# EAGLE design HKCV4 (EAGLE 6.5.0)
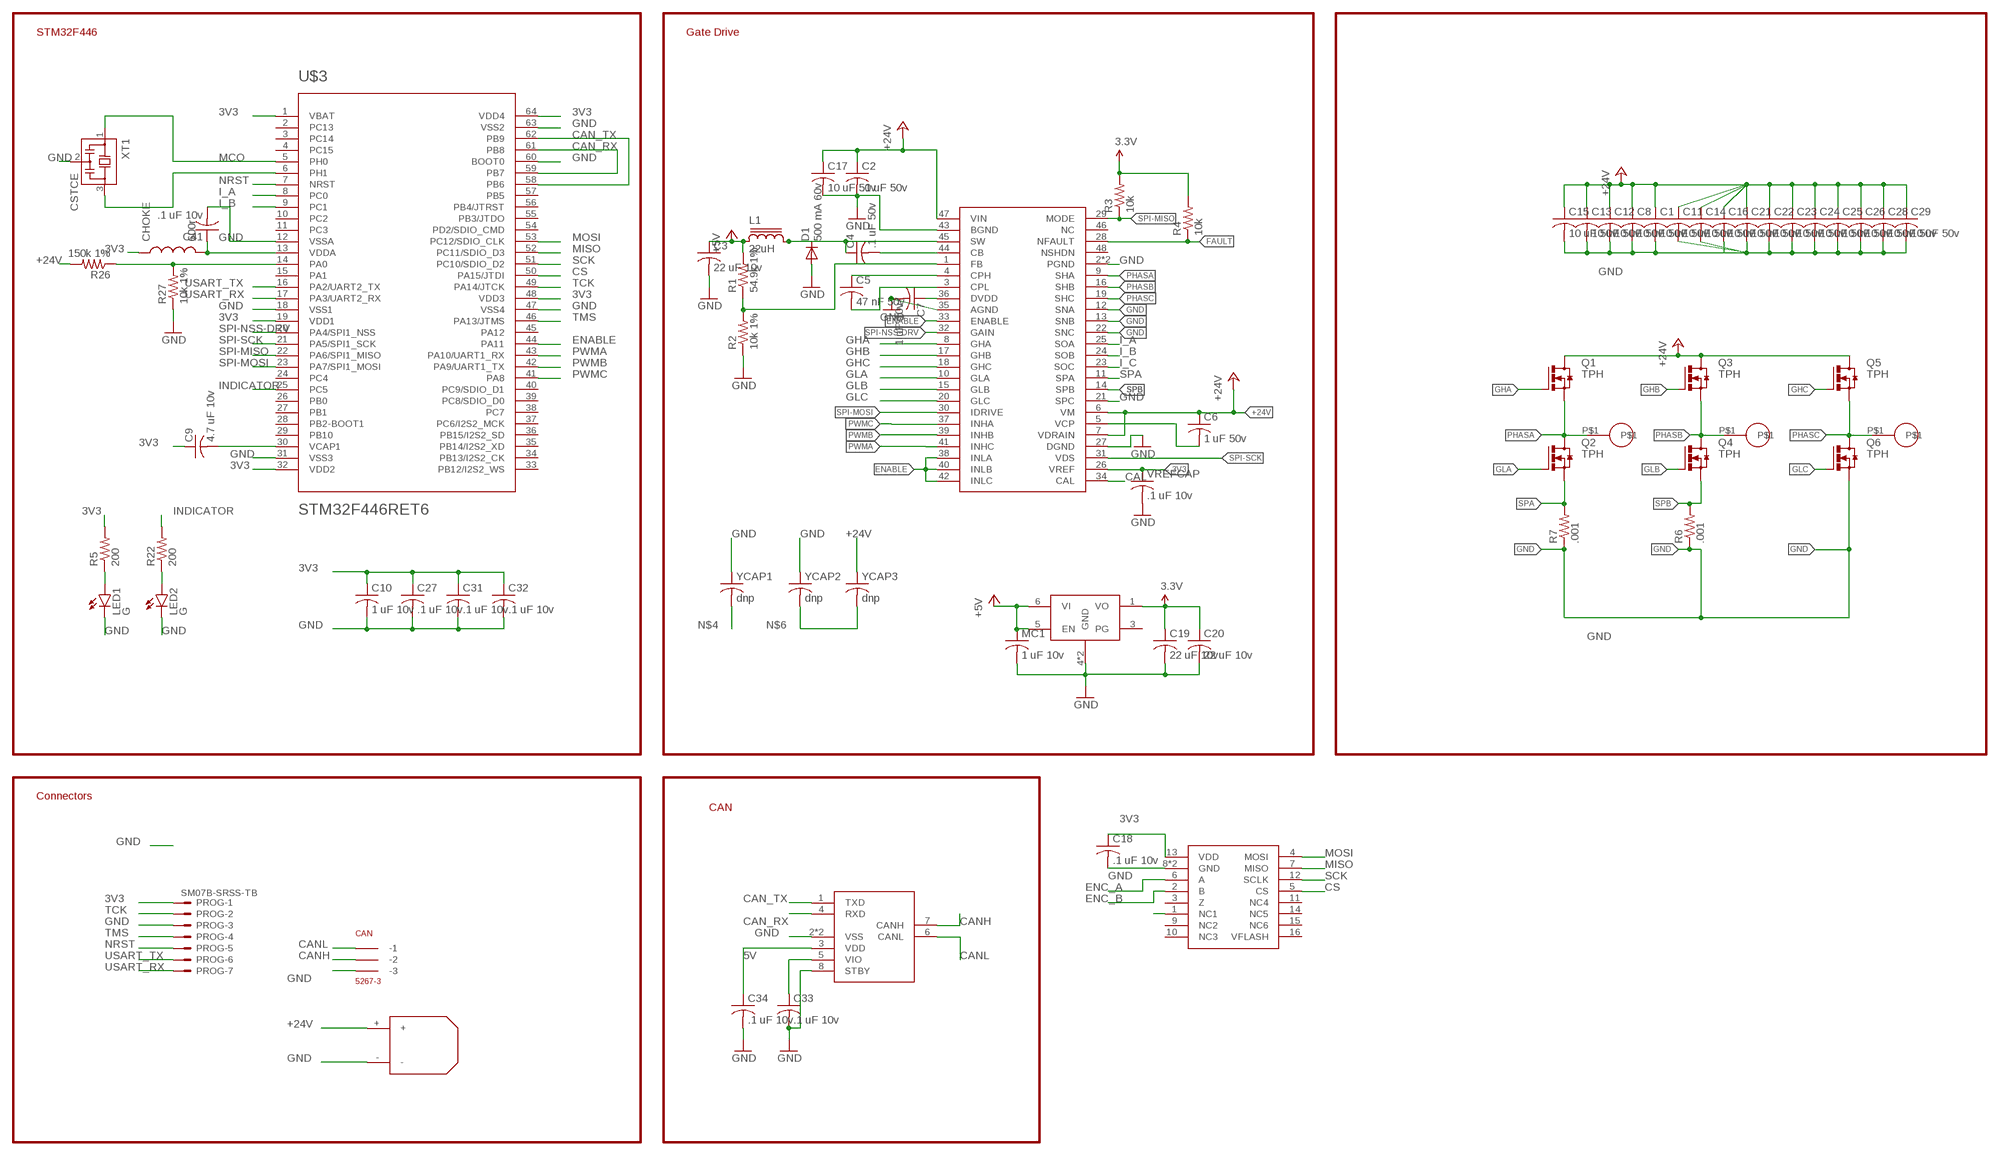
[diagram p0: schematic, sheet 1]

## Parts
C1  10 uF 50v  C-USC1206K  [C1206K]
C2  .1 uF 50v  C-USC0603K  [C0603K]
C3  22 uF 10v  C-USC0603K  [C0603K]
C4  .1 uF 50v  C-USC0603K  [C0603K]
C5  47 nF 50v  C-USC0402K  [C0402K]
C6  1 uF 50v  C-USC0603K  [C0603K]
C7  1 uF 10v  C-USC0402K  [C0402K]
C8  10 uF 50v  C-USC1206K  [C1206K]
C9  4.7 uF 10v  C-USC0402K  [C0402K]
C10  1 uF 10v  C-USC0402K  [C0402K]
C11  10 uF 50v  C-USC1206K  [C1206K]
C12  10 uF 50v  C-USC1206K  [C1206K]
C13  10 uF 50v  C-USC1206K  [C1206K]
C14  10 uF 50v  C-USC1206K  [C1206K]
C15  10 uF 50v  C-USC1206K  [C1206K]
C16  10 uF 50v  C-USC1206K  [C1206K]
C17  10 uF 50v  C-USC1206K  [C1206K]
C18  .1 uF 10v  C-USC0402K  [C0402K]
C19  22 uF 10v  C-USC0603K  [C0603K]
C20  22 uF 10v  C-USC0603K  [C0603K]
C21  10 uF 50v  C-USC1206K  [C1206K]
C22  10 uF 50v  C-USC1206K  [C1206K]
C23  10 uF 50v  C-USC1206K  [C1206K]
C24  10 uF 50v  C-USC1206K  [C1206K]
C25  10 uF 50v  C-USC1206K  [C1206K]
C26  10 uF 50v  C-USC1206K  [C1206K]
C27  .1 uF 10v  C-USC0402K  [C0402K]
C28  10 uF 50v  C-USC1206K  [C1206K]
C29  10 uF 50v  C-USC1206K  [C1206K]
C31  .1 uF 10v  C-USC0402K  [C0402K]
C32  .1 uF 10v  C-USC0402K  [C0402K]
C33  .1 uF 10v  C-USC0402K  [C0402K]
C34  .1 uF 10v  C-USC0402K  [C0402K]
C41  .1 uF 10v  C-USC0402K  [C0402K]
CAN  5267-3  [5267-3]
CHOKE  600r  INDUCTOR0603  [0603]
D1  500 mA 60v  DIODE-SOD123  [SOD123]
L1  22uH  SDR0302  [SDR0302]
LDFM33PUR  LDFM  [DFN6-3X3]
LED1  G  LED0603  [LED-0603]
LED2  G  LED0603  [LED-0603]
MC1  1 uF 10v  C-USC0402K  [C0402K]
PROG  SM07B-SRSS-TB  [SM07B-SRSS-TB]
Q1  TPH  [TRANS_TPH5900CNH,L1Q]
Q2  TPH  [TRANS_TPH5900CNH,L1Q]
Q3  TPH  [TRANS_TPH5900CNH,L1Q]
Q4  TPH  [TRANS_TPH5900CNH,L1Q]
Q5  TPH  [TRANS_TPH5900CNH,L1Q]
Q6  TPH  [TRANS_TPH5900CNH,L1Q]
R1  54.9k 1%  R-US_R0402  [R0402]
R2  10k 1%  R-US_R0402  [R0402]
R3  10k  R-US_R0402  [R0402]
R4  10k  R-US_R0402  [R0402]
R5  200  R-US_R0402  [R0402]
R6  .001  R-US_R1210  [R1210]
R7  .001  R-US_R1210  [R1210]
R22  200  R-US_R0402  [R0402]
R26  150k 1%  R-US_R0402  [R0402]
R27  10k 1%  R-US_R0402  [R0402]
U$1  DRV8323RH  [QFN50P700X700X90-49N]
U$2  18_AWG_PAD  [18_AWG_PAD]
U$3  STM32F446RET6  [TQFP64]
U$4  18_AWG_PAD  [18_AWG_PAD]
U$5  18_AWG_PAD  [18_AWG_PAD]
U$6  MCP2542  [TDFN]
U$9  XT30  [XT30_HORIZONTAL]
U$11  MA700  [QFN16]
VREFCAP  .1 uF 10v  C-USC0402K  [C0402K]
XT1  CSTCE  [CSTCE]
YCAP1  dnp  C-USC0402K  [C0402K]
YCAP2  dnp  C-USC0402K  [C0402K]
YCAP3  dnp  C-USC0402K  [C0402K]

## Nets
3V3: C9.1 C10.1 C18.1 C19.1 C20.1 C27.1 C31.1 C32.1 C33.1 CHOKE.1 LDFM33PUR.1(VO) PROG.1 R3.2 R4.2 R5.2 U$1.26(VREF) U$3.1(VBAT) U$3.19(VDD1) U$3.32(VDD2) U$3.48(VDD3) U$3.64(VDD4) U$6.5(VIO) U$11.13(VDD) VREFCAP.1 ; supply symbol labelled 3.3V
5V: C3.1 C34.1 L1.1 LDFM33PUR.5(EN) LDFM33PUR.6(VI) MC1.1 R1.2 U$6.3(VDD) ; supply symbol labelled +5V
+24V: C1.1 C2.1 C6.1 C8.1 C11.1 C12.1 C13.1 C14.1 C15.1 C16.1 C17.1 C21.1 C22.1 C23.1 C24.1 C25.1 C26.1 C28.1 C29.1 Q1.5(D) Q1.6(D) Q1.7(D) Q1.8(D) Q1.EP(D) Q3.5(D) Q3.6(D) Q3.7(D) Q3.8(D) Q3.EP(D) Q5.5(D) Q5.6(D) Q5.7(D) Q5.8(D) Q5.EP(D) R26.2 U$1.6(VM) U$1.7(VDRAIN) U$1.47(VIN) U$9.+ YCAP3.1
BOOT: C4.2 U$1.44(CB)
CAL: U$1.34(CAL)
CAN_RX: U$3.59(PB7) U$3.61(PB8) U$6.4(RXD)
CAN_TX: U$3.58(PB6) U$3.62(PB9) U$6.1(TXD)
CANH: CAN.P$2(-2) U$6.7(CANH)
CANL: CAN.P$1(-1) U$6.6(CANL)
CPH: C5.1 U$1.4(CPH)
CPL: C5.2 U$1.3(CPL)
CS: U$3.50(PA15/JTDI) U$11.5(CS)
DEVICE3.3: C7.1 U$1.36(DVDD)
ENABLE: U$1.33(ENABLE) U$1.38(INLA) U$1.40(INLB) U$1.42(INLC) U$3.44(PA11)
ENC_A: U$11.6(A)
ENC_B: U$11.2(B)
FAULT: R4.1 U$1.28(NFAULT)
FB: R1.1 R2.2 U$1.1(FB)
GHA: Q1.4(G) U$1.8(GHA)
GHB: Q3.4(G) U$1.17(GHB)
GHC: Q5.4(G) U$1.18(GHC)
GLA: Q2.4(G) U$1.10(GLA)
GLB: Q4.4(G) U$1.15(GLB)
GLC: Q6.4(G) U$1.20(GLC)
GND: C1.2 C2.2 C3.2 C7.2 C8.2 C10.2 C11.2 C12.2 C13.2 C14.2 C15.2 C16.2 C17.2 C18.2 C19.2 C20.2 C21.2 C22.2 C23.2 C24.2 C25.2 C26.2 C27.2 C28.2 C29.2 C31.2 C32.2 C33.2 C34.2 C41.2 CAN.P$3(-3) D1.A LDFM33PUR.4(GND) LDFM33PUR.EXP(GND) LED1.C LED2.C MC1.2 PROG.3 Q6.1(S) Q6.2(S) Q6.3(S) R2.1 R6.1 R7.1 R27.1 U$1.2(PGND) U$1.12(SNA) U$1.13(SNB) U$1.21(SPC) U$1.22(SNC) U$1.27(DGND) U$1.35(AGND) U$1.43(BGND) U$1.49(PGND) U$3.12(VSSA) U$3.18(VSS1) U$3.31(VSS3) U$3.47(VSS4) U$3.60(BOOT0) U$3.63(VSS2) U$6.2(VSS) U$6.8(STBY) U$6.9(VSS) U$9.- U$11.8(GND) U$11.TH(GND) VREFCAP.2 XT1.2 YCAP1.1 YCAP2.1
I_A: U$1.25(SOA) U$3.8(PC0)
I_B: U$1.24(SOB) U$3.9(PC1)
I_C: U$1.23(SOC)
INDICATOR: R22.2 U$3.25(PC5)
MCO: U$3.5(PH0) XT1.1
MISO: U$3.52(PC11/SDIO_D3) U$11.7(MISO)
MOSI: U$3.53(PC12/SDIO_CLK) U$11.4(MOSI)
N$1: LED1.A R5.1
N$2: C41.1 CHOKE.2 U$3.13(VDDA)
N$3: C9.2 U$3.30(VCAP1)
N$4: YCAP1.2
N$6: YCAP2.2 YCAP3.2
N$9: U$11.1(NC1)
N$24: R26.1 R27.2 U$3.14(PA0)
N$28: LED2.A R22.1
N$30: U$3.6(PH1) XT1.3
NRST: PROG.5 U$3.7(NRST)
PHASA: Q1.1(S) Q1.2(S) Q1.3(S) Q2.5(D) Q2.6(D) Q2.7(D) Q2.8(D) Q2.EP(D) U$1.9(SHA) U$4.P$1
PHASB: Q3.1(S) Q3.2(S) Q3.3(S) Q4.5(D) Q4.6(D) Q4.7(D) Q4.8(D) Q4.EP(D) U$1.16(SHB) U$2.P$1
PHASC: Q5.1(S) Q5.2(S) Q5.3(S) Q6.5(D) Q6.6(D) Q6.7(D) Q6.8(D) Q6.EP(D) U$1.19(SHC) U$5.P$1
PWMA: U$1.41(INHC) U$3.43(PA10/UART1_RX)
PWMB: U$1.39(INHB) U$3.42(PA9/UART1_TX)
PWMC: U$1.37(INHA) U$3.41(PA8)
SCK: U$3.51(PC10/SDIO_D2) U$11.12(SCLK)
SPA: Q2.1(S) Q2.2(S) Q2.3(S) R7.2 U$1.11(SPA)
SPB: Q4.1(S) Q4.2(S) Q4.3(S) R6.2 U$1.14(SPB)
SPI-MISO: R3.1 U$1.29(MODE) U$3.22(PA6/SPI1_MISO)
SPI-MOSI: U$1.30(IDRIVE) U$3.23(PA7/SPI1_MOSI)
SPI-NSS-DRV: U$1.32(GAIN) U$3.20(PA4/SPI1_NSS)
SPI-SCK: U$1.31(VDS) U$3.21(PA5/SPI1_SCK)
SW: C4.1 D1.C L1.2 U$1.45(SW)
TCK: PROG.2 U$3.49(PA14/JTCK)
TMS: PROG.4 U$3.46(PA13/JTMS)
USART_RX: PROG.7 U$3.17(PA3/UART2_RX)
USART_TX: PROG.6 U$3.16(PA2/UART2_TX)
VCP: C6.2 U$1.5(VCP)
Unconnected: LDFM33PUR.3(PG) U$1.46(NC) U$1.48(NSHDN) U$3.2(PC13) U$3.3(PC14) U$3.4(PC15) U$3.10(PC2) U$3.11(PC3) U$3.15(PA1) U$3.24(PC4) U$3.26(PB0) U$3.27(PB1) U$3.28(PB2-BOOT1) U$3.29(PB10) U$3.33(PB12/I2S2_WS) U$3.34(PB13/I2S2_CK) U$3.35(PB14/I2S2_XD) U$3.36(PB15/I2S2_SD) U$3.37(PC6/I2S2_MCK) U$3.38(PC7) U$3.39(PC8/SDIO_D0) U$3.40(PC9/SDIO_D1) U$3.45(PA12) U$3.54(PD2/SDIO_CMD) U$3.55(PB3/JTDO) U$3.56(PB4/JTRST) U$3.57(PB5) U$11.3(Z) U$11.9(NC2) U$11.10(NC3) U$11.11(NC4) U$11.14(NC5) U$11.15(NC6) U$11.16(VFLASH)

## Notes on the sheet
- STM32F446 | Gate Drive
- Connectors
- CAN

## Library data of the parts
C1-C29 C31-C34 C41 MC1 VREFCAP YCAP1-YCAP3 = rcl:C-US: CAPACITOR, American symbol
CAN = con-molex-spox:5267-3
CHOKE = SparkFun-Passives:INDUCTOR: Inductors
D1 = diode:DIODE-: DIODE
L1 = inductor-bourns:SDR0302: POWER INDUCTOR
LDFM33PUR = BenLibrary:LDFM
LED1 LED2 = SparkFun-LED:LED: LEDs
PROG = con-jst2:?M07B-SRSS-TB: Disconnectable Crimp style connector, 1.0mm pitch 7 contacts
Q1-Q6 = transistor-power:TPH
R1-R7 R22 R26 R27 = rcl:R-US_: RESISTOR, American symbol
U$1 = BenLibrary:DRV8323RH
U$2 U$4 U$5 = BenLibrary:18_AWG_PAD
U$3 = BenLibrary:STM32F446RET6: ARM DSP Chip used on the WAV Trigger board.
U$6 = BenLibrary:MCP2542
U$9 = Ben_Library:XT30
U$11 = BenLibrary:MA700
XT1 = sc_usercreated:CSTCE

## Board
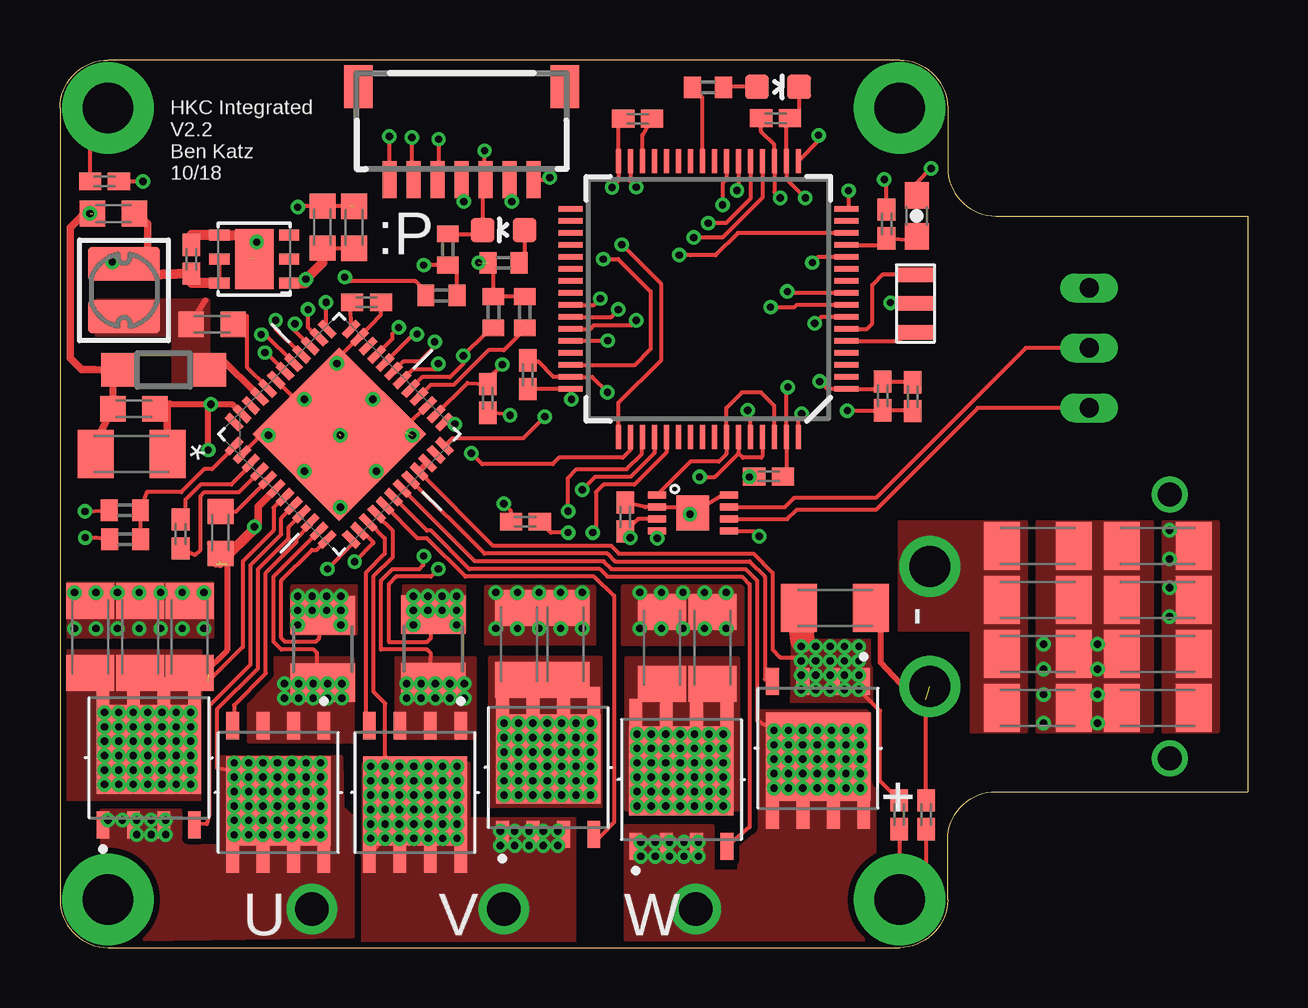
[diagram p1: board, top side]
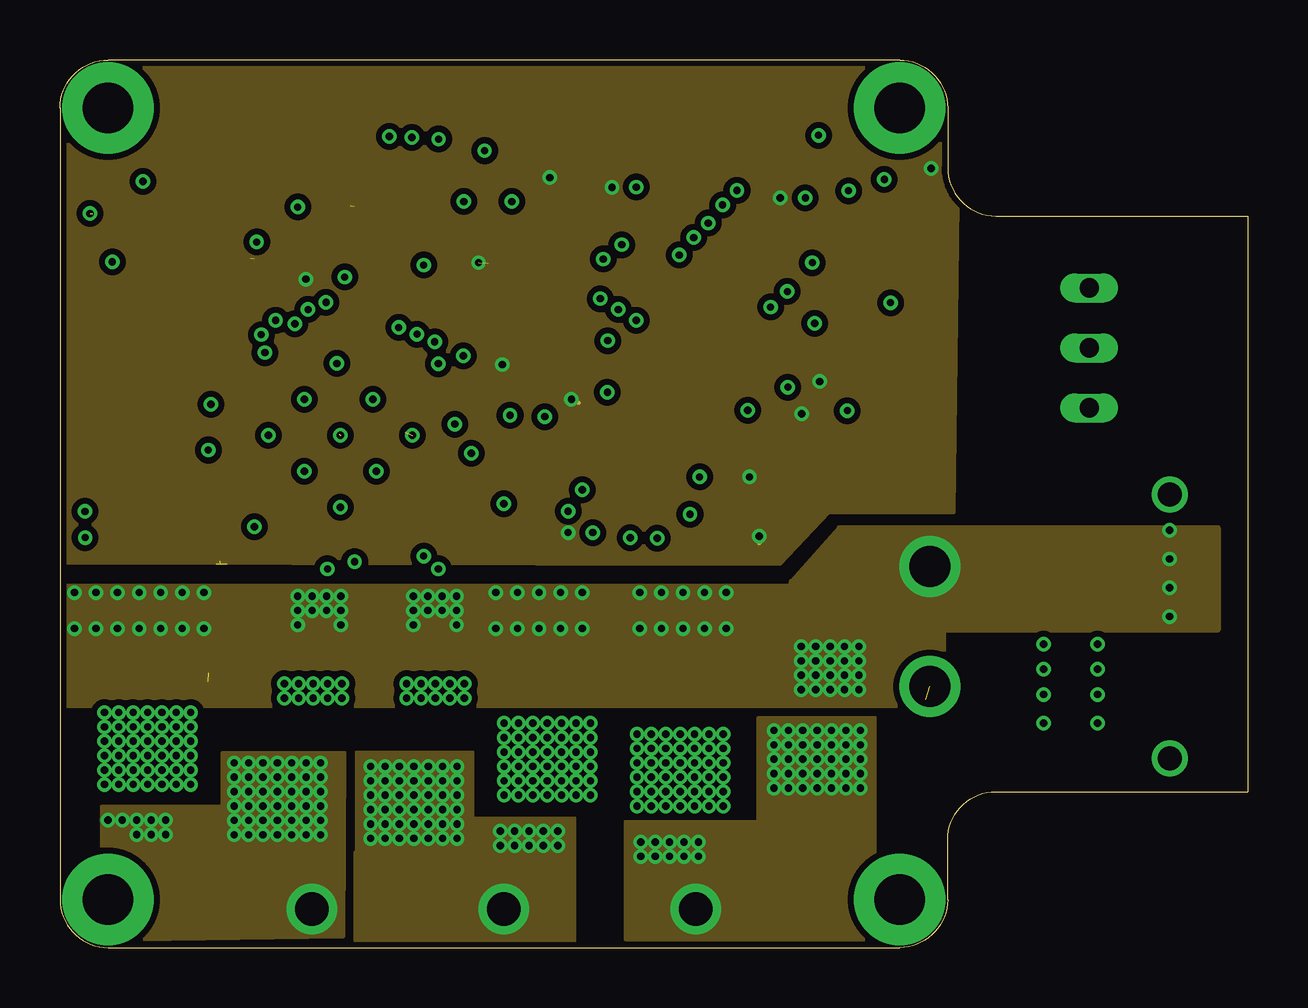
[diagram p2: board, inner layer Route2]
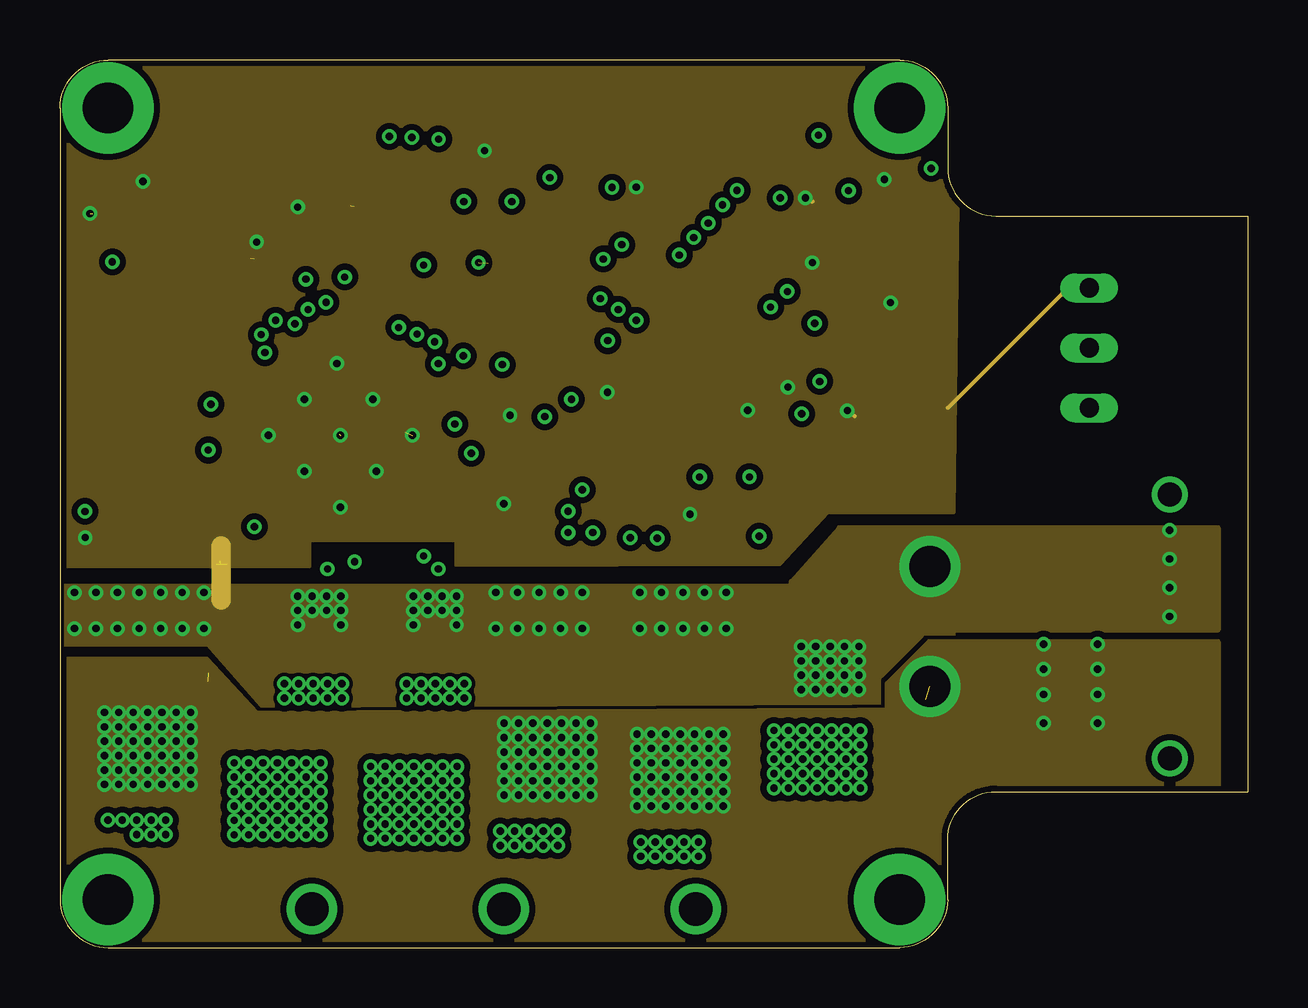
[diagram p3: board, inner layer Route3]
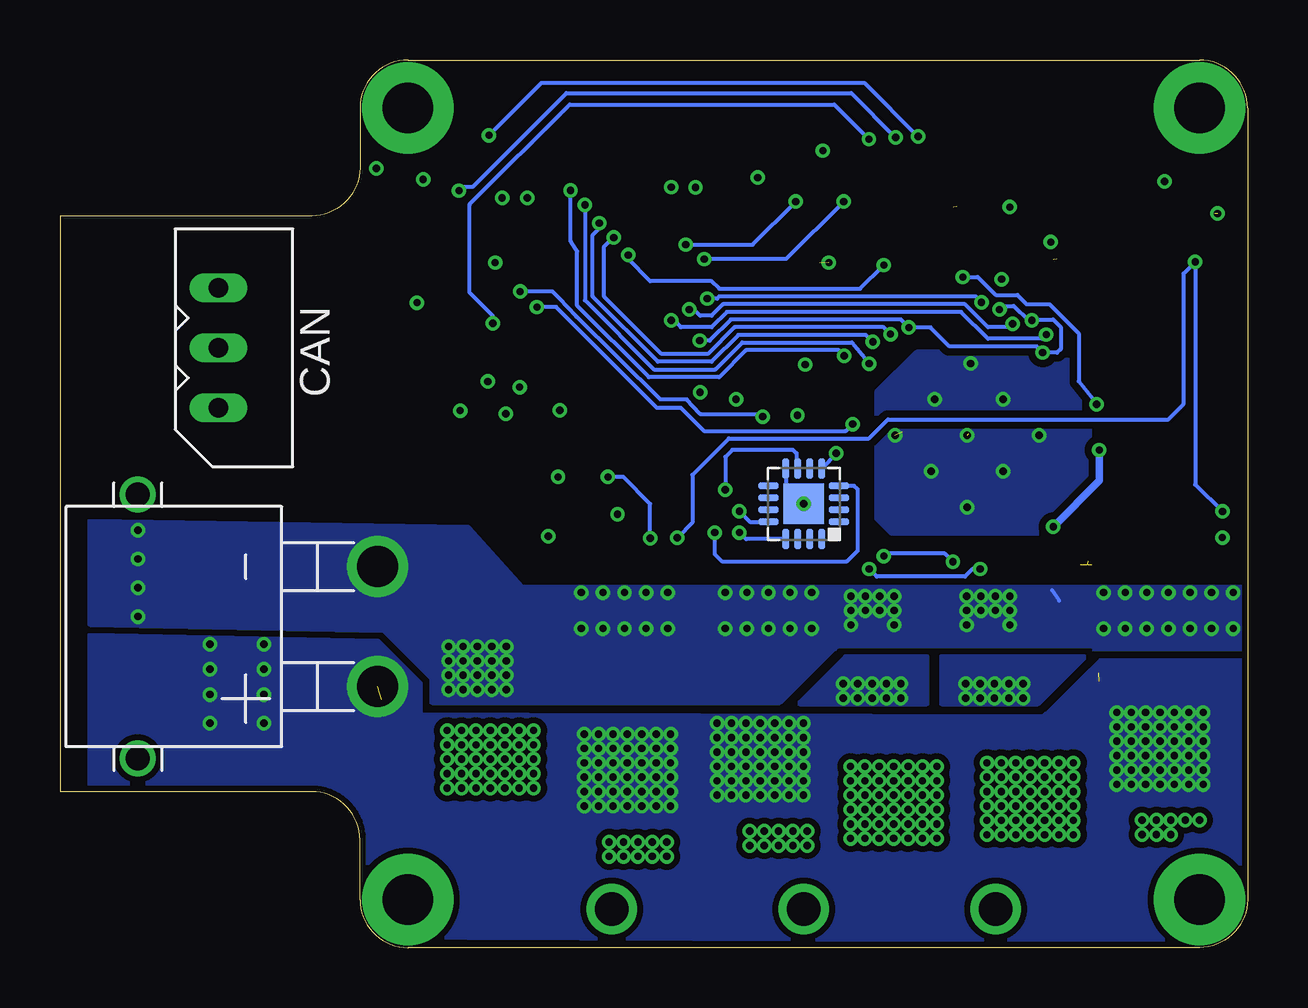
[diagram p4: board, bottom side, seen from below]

Size 49.5 x 37 mm. Coordinates in mm from the lower left corner, seen from the top.
Outline: 2,0 35,0 arc90 37,2 37,4.5 arc-90 39,6.5 49.5,6.5 49.5,30.5 39,30.5 arc-90 37,32.5 37,35 arc90 35,37 2,37 arc90 0,35 0,2 arc90 2,0
Copper layers (1*2+3*16): Top 0.035mm / dielectric 1.5mm / Route2 0.035mm / dielectric 0.15mm / Route3 0.035mm / dielectric 0.2mm / Bottom 0.035mm
Design rules "default *": minimum track width 6mil, minimum drill 0.3mm, track to track 6mil, track to pad 6mil, pad to pad 6mil, via to via 6mil, smd to smd 6mil, copper to edge 6mil, drill to drill 6mil, minimum pad ring 0.15mm, minimum via ring 0.15mm, stop-mask expansion 4mil, vias tented up to drill 12mil, thermal gap 10mil

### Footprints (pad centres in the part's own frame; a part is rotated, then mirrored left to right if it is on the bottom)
C1206K = smd 1.5 x 2: 1 -1.5,0; 2 1.5,0
C0603K = smd 1.05 x 1.08: 1 -0.875,0; 2 0.875,0
C0402K = smd 0.925 x 0.74: 1 -0.6,0; 2 0.6,0
5267-3 = drill 0.8 long: P$1 0,0; P$2 2.5,0; P$3 5,0
0603 = smd 1.1 x 1: 1 -0.85,0; 2 0.85,0
SOD123 = smd 1.4 x 1.4: A 1.9,0; C -1.9,0
SDR0302 = smd 3 x 1.4: 1 0,1.1; 2 0,-1.1
DFN6-3X3 = smd 0.85 x 0.45: 1 -1.45,1; 2 -1.45,0; 3 -1.45,-1; 4 1.45,-1; 5 1.45,0; 6 1.45,1 | smd 1.6 x 2.5: EXP 0,0
LED-0603 = smd 1 x 1: A 0,-0.877; C 0,0.877
SM07B-SRSS-TB = smd 0.6 x 1.55: 1 -3,2.975; 2 -2,2.975; 3 -1,2.975; 4 0,2.975; 5 1,2.975; 6 2,2.975; 7 3,2.975 | smd 1.2 x 1.8: FIT@1 -4.3,-0.9; FIT@2 4.3,-0.9
TRANS_TPH5900CNH,L1Q = smd 1.13 x 0.53: 1 -2.79,1.905; 2 -2.79,0.635; 3 -2.79,-0.635; 4 -2.79,-1.905 | smd 1.33 x 0.53: 5 2.69,-1.905; 6 2.69,-0.635; 7 2.69,0.635; 8 2.69,1.905 | smd 3.7 x 4.35: EP 0.35,0
R0402 = smd 0.7 x 0.9: 1 -0.65,0; 2 0.65,0
R1210 = smd 1.6 x 2.7: 1 -1.4,0; 2 1.4,0
QFN50P700X700X90-49N = smd 0.813 x 0.305: 1 -3.454,2.743; 2 -3.454,2.261; 3 -3.454,1.753; 4 -3.454,1.245; 5 -3.454,0.762; 6 -3.454,0.254; 7 -3.454,-0.254; 8 -3.454,-0.762; 9 -3.454,-1.245; 10 -3.454,-1.753; 11 -3.454,-2.261; 12 -3.454,-2.743; 25 3.454,-2.743; 26 3.454,-2.261; 27 3.454,-1.753; 28 3.454,-1.245; 29 3.454,-0.762; 30 3.454,-0.254; 31 3.454,0.254; 32 3.454,0.762; 33 3.454,1.245; 34 3.454,1.753; 35 3.454,2.261; 36 3.454,2.743 | smd 0.305 x 0.813: 13 -2.743,-3.454; 14 -2.261,-3.454; 15 -1.753,-3.454; 16 -1.245,-3.454; 17 -0.762,-3.454; 18 -0.254,-3.454; 19 0.254,-3.454; 20 0.762,-3.454; 21 1.245,-3.454; 22 1.753,-3.454; 23 2.261,-3.454; 24 2.743,-3.454; 37 2.743,3.454; 38 2.261,3.454; 39 1.753,3.454; 40 1.245,3.454; 41 0.762,3.454; 42 0.254,3.454; 43 -0.254,3.454; 44 -0.762,3.454; 45 -1.245,3.454; 46 -1.753,3.454; 47 -2.261,3.454; 48 -2.743,3.454 | smd 5.105 x 5.105: 49 0,0
18_AWG_PAD = drill 1.4: P$1 0,0
TQFP64 = smd 0.22 x 1: 1 -3.75,-5.75; 2 -3.25,-5.75; 3 -2.75,-5.75; 4 -2.25,-5.75; 5 -1.75,-5.75; 6 -1.25,-5.75; 7 -0.75,-5.75; 8 -0.25,-5.75; 9 0.25,-5.75; 10 0.75,-5.75; 11 1.25,-5.75; 12 1.75,-5.75; 13 2.25,-5.75; 14 2.75,-5.75; 15 3.25,-5.75; 16 3.75,-5.75; 33 3.75,5.75; 34 3.25,5.75; 35 2.75,5.75; 36 2.25,5.75; 37 1.75,5.75; 38 1.25,5.75; 39 0.75,5.75; 40 0.25,5.75; 41 -0.25,5.75; 42 -0.75,5.75; 43 -1.25,5.75; 44 -1.75,5.75; 45 -2.25,5.75; 46 -2.75,5.75; 47 -3.25,5.75; 48 -3.75,5.75 | smd 1 x 0.22: 17 5.75,-3.75; 18 5.75,-3.25; 19 5.75,-2.75; 20 5.75,-2.25; 21 5.75,-1.75; 22 5.75,-1.25; 23 5.75,-0.75; 24 5.75,-0.25; 25 5.75,0.25; 26 5.75,0.75; 27 5.75,1.25; 28 5.75,1.75; 29 5.75,2.25; 30 5.75,2.75; 31 5.75,3.25; 32 5.75,3.75; 49 -5.75,3.75; 50 -5.75,3.25; 51 -5.75,2.75; 52 -5.75,2.25; 53 -5.75,1.75; 54 -5.75,1.25; 55 -5.75,0.75; 56 -5.75,0.25; 57 -5.75,-0.25; 58 -5.75,-0.75; 59 -5.75,-1.25; 60 -5.75,-1.75; 61 -5.75,-2.25; 62 -5.75,-2.75; 63 -5.75,-3.25; 64 -5.75,-3.75
TDFN = smd 0.3 x 0.75: 1 0,-3; 2 0.5,-3; 3 1,-3; 4 1.5,-3; 5 1.5,0; 6 1,0; 7 0.5,0; 8 0,0 | smd 1.46 x 1.36: 9 0.75,-1.5
XT30_HORIZONTAL = drill 1.7: + -2.5,0; - 2.5,0 | drill 1: P$3 5.5,10; P$4 -5.5,10
QFN16 = smd 0.85 x 0.3: 1 -1.475,0.75; 2 -1.475,0.25; 3 -1.475,-0.25; 4 -1.475,-0.75; 9 1.475,-0.75; 10 1.475,-0.25; 11 1.475,0.25; 12 1.475,0.75 | smd 0.3 x 0.85: 5 -0.75,-1.475; 6 -0.25,-1.475; 7 0.25,-1.475; 8 0.75,-1.475; 13 0.75,1.475; 14 0.25,1.475; 15 -0.25,1.475; 16 -0.75,1.475 | smd 1.7 x 1.7: TH 0,0
CSTCE = smd 0.6 x 1.6: 1 -1.2,0; 2 0,0; 3 1.2,0

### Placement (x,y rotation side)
C1  19.13,12.65 90 top
C2  3.08,22.46 180 top
C3  2.23,30.59 180 top
C4  6.34,25.98 0 top
C5  5.03,17.24 90 top
C6  6.69,17.3 90 top
C7  12.78,26.9 0 top
C8  5.4,12.95 90 top
C9  24.08,34.55 0 top
C10  35.54,22.96 270 top
C11  3.35,12.95 90 top
C12  27.19,12.5 90 top
C13  25.09,12.5 90 top
C14  21.07,12.65 90 top
C15  1.25,12.95 90 top
C16  32.31,14.15 180 top
C17  2.98,20.58 180 top
C18  19.4,17.75 180 top
C19  10.94,30.03 90 top
C20  12.26,30.02 90 top
C21  45.75,14.5 0 top
C22  40.75,16.75 180 top
C23  40.75,14.5 180 top
C24  40.75,12.25 180 top
C25  40.75,10 180 top
C26  45.75,16.75 0 top
C27  29.83,34.57 0 top
C28  45.75,12.25 0 top
C29  45.75,10 0 top
C31  34.29,23 270 top
C32  19.5,23.88 90 top
C33  29.54,19.64 0 top
C34  23.56,17.95 90 top
C41  34.45,30.16 90 top
CAN  42.9,22.5 90 bottom
CHOKE  35.71,30.5 270 top
D1  4.32,24.08 180 top
L1  2.67,27.4 0 top
LDFM33PUR  8.1,28.7 180 top
LED1  18.49,29.91 90 top
LED2  29.93,35.88 270 top
MC1  5.48,28.69 90 top
PROG  16.74,34.98 180 top
Q1  3.7,7.91 90 top
Q2  9.1,6.46 270 top
Q3  20.35,7.51 90 top
Q4  14.8,6.46 270 top
Q5  25.9,7.01 90 top
Q6  31.6,8.31 270 top
R1  2.7,18.23 180 top
R2  2.72,17.02 0 top
R3  18.07,26.48 90 top
R4  19.38,26.48 90 top
R5  18.49,28.54 180 top
R6  15.56,12.47 270 top
R7  10.96,12.45 270 top
R22  27.01,35.85 180 top
R26  15.9,27.18 180 top
R27  16.17,29.1 270 top
U$1  11.64,21.4 45 top
U$2  18.5,1.6 0 top
U$3  27.03,27.04 90 top
U$4  10.5,1.6 0 top
U$5  26.5,1.6 0 top
U$6  27.88,18.86 270 top
U$9  36.26,13.38 90 bottom
U$11  18.5,18.5 180 bottom
VREFCAP  17.83,22.89 270 top
XT1  35.66,26.85 90 top
YCAP1  1.86,31.94 180 top
YCAP2  34.98,5.54 270 top
YCAP3  36.1,5.54 270 top

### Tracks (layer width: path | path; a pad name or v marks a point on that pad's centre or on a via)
3V3  (via drill 0.3)  (1 unrouted)
  Top 0.16: R4.2 R3.2 18.07,28.31 R5.2 | v21.32,22.85 21.28,22.89 U$3.48 C32.1 | U$3.64 30.78,22.11 v30.92,22.25 | v31.67,23.6 31.98,23.29 U$3.1 34.29,23.29 C31.1 35.54,23.6 C10.1 | v30.02,31.25 29.78,31.49 U$3.19 29.78,33.46 29.22,34.02 C27.1 | U$6.5 28.94,17.36 v29.15,17.15 | v21.18,17.3 20.45,17.3 C18.1 | CHOKE.1 35.71,31.88 v36.31,32.48 | 28.72,19.62 v28.74,19.62 28.76,19.64 C33.1 | C9.1 23.28,34.31 U$3.32 23.28,31.96 v23.01,31.69 | U$1.26 16.98,23.54 VREFCAP.1 17.83,23.69 v18.44,24.3 | C20.1 C19.1 | PROG.1 20.42,32.01 v20.42,32.1
  Top 0.406: LDFM33PUR.1 10.25,27.7 v10.25,27.86 10.94,28.55 C19.1
  Route2 0.16: v21.32,22.85 21.47,22.85 21.62,22.7 | v30.92,22.25 31.07,22.4 | v31.67,23.6 31.67,23.75 | v30.02,31.25 30.17,31.1 | v29.15,17.15 29.15,16.85
  Bottom 0.16: U$11.13 20.91,17.02 v21.18,17.3
  other vias: 17.45,28.55
  pour Route2 (isolate 0.254, no thermals): -0.5,16.05 30,16 32.05,18.15 37.25,18.15 37.5,37.5 -0.5,37.5
5V  (via drill 0.3)
  Top 0.16: L1.1 2.26,28.5 v2.18,28.58 | v1.04,18.18 1.15,18.18 R1.2 | v23.77,17.08 23.77,17.3 C34.1 23.59,17.35 24.1,17.86 U$6.3 | LDFM33PUR.6 LDFM33PUR.5
  Top 0.2: 3.65,28.5 3.25,28.9
  Top 0.26: 3.7,28.95 3.25,28.9 L1.1
  Top 0.305: C3.1 3.65,30.17 3.65,28.5
  Top 0.406: 3.65,28.5 3.65,28.04 MC1.1 5.48,27.7 LDFM33PUR.6
  Bottom 0.16: v1.04,18.18 2.18,19.3 v2.18,28.58 2.66,28.1 2.66,22.66 3.3,22.02 14.98,22.02 15.78,21.22 21.62,21.22 23.14,19.7 23.14,17.71 v23.77,17.08
+24V  (via drill 0.3, 0.3 pad 0.25)  (5 unrouted)
  Top 0.16: Q1.5 5.36,7.71 | C6.1 6.2,16.84 | 6.2,11.45 6.02,11.45 C8.1 | 6.18,11.09 7.62,12.53 7.62,16.1 8.9,17.38 8.9,18.34 9.34,18.78 U$1.7 | R26.2 15.25,27.35 14.82,27.78 12.04,27.78 v11.87,27.95 | YCAP3.1 36.1,10.35 35.6,10.4
  Top 0.25: 6.96,15.96 6.96,16.26
  Top 0.26: 6.52,16.28 6.5,15.96 | v6.29,22.65 7.17,22.65 U$1.47 | C2.1 4.58,22.65 v6.29,22.65 | C16.1 33.65,13.55 34.2,13.25 34.2,11.9 35.6,10.4 | 6.96,15.96 6.96,12.39 6.02,11.45 | v6.18,20.74 6.18,22.54 v6.29,22.65
  Top 0.305: C17.1 4.46,22.53 4.58,22.65 | U$1.6 8.26,18.38 8.26,17.54 6.68,15.96 | v8.1,17.54 6.66,16.11 C6.1
  Bottom 0.16: v6.29,22.65 7.04,23.6 7.04,25.6 8.26,26.82 9.21,26.82 9.59,27.2 10.49,27.2 11.24,27.95 v11.87,27.95
  Bottom 0.305: v6.18,20.74 6.18,19.46 v8.1,17.54
  other vias: 27.65,8.3 27.65,7.7 27.65,7.1 27.65,6.5 27.65,5.9 24.05,8.3 24.05,7.7 24.05,7.1 24.05,6.5 24.05,5.9 24.65,8.3 24.65,7.7 24.65,7.1 24.65,6.5 24.65,5.9 25.25,8.3 25.25,7.7 25.25,7.1 25.25,6.5 25.25,5.9 25.85,8.3 25.85,7.7 25.85,7.1 25.85,6.5 25.85,5.9 26.45,8.3 26.45,7.7 26.45,7.1 26.45,6.5 26.45,5.9 27.05,8.3 27.05,7.7 27.05,7.1 27.05,6.5 27.05,5.9 18.51,8.75 18.51,8.15 18.51,7.55 18.51,6.95 18.51,6.35 19.11,8.75 19.11,8.15 19.11,7.55 19.11,6.95 19.11,6.35 19.71,8.75 19.71,8.15 19.71,7.55 19.71,6.95 19.71,6.35 20.31,8.75 20.31,8.15 20.31,7.55 20.31,6.95 20.31,6.35 20.91,8.75 20.91,8.15 20.91,7.55 20.91,6.95 20.91,6.35 21.51,8.75 21.51,8.15 21.51,7.55 21.51,6.95 21.51,6.35 22.11,8.75 22.11,8.15 22.11,7.55 22.11,6.95 22.11,6.35 1.85,9.2 1.85,8.6 1.85,8 1.85,7.4 1.85,6.8 2.45,9.2 2.45,8.6 2.45,8 2.45,7.4 2.45,6.8 3.05,9.2 3.05,8.6 3.05,8 3.05,7.4 3.05,6.8 3.65,9.2 3.65,8.6 3.65,8 3.65,7.4 3.65,6.8 4.25,9.2 4.25,8.6 4.25,8 4.25,7.4 4.25,6.8 4.85,9.2 4.85,8.6 4.85,8 4.85,7.4 4.85,6.8 5.45,9.2 5.45,8.6 5.45,8 5.45,7.4 5.45,6.8 24.05,8.9 24.65,8.9 25.25,8.9 25.85,8.9 26.45,8.9 27.05,8.9 27.65,8.9 18.51,9.35 19.11,9.35 19.71,9.35 20.31,9.35 20.91,9.35 21.51,9.35 22.11,9.35 1.85,9.8 2.45,9.8 3.05,9.8 3.65,9.8 4.25,9.8 4.85,9.8 5.45,9.8 43.25,9.35 43.25,10.55 43.25,11.6 43.25,12.65 41,12.65 41,11.6 41,10.55 41,9.35
  pour Bottom (isolate 0.254, rank 2, no thermals): 37.1,9.75 8.52,9.65 6.12,12 -0.2,12 -0.35,0.25 37.25,0.4
  pour Top (no thermals): 23.61,12.07 28.26,12.07 28.26,5.75 23.61,5.75
  pour Top (no thermals): 22.56,5.9 22.56,12.07 17.91,12.07 17.91,5.9
  pour Top (isolate 0.254, no thermals): -0.1,6.2 5.87,6.2 5.87,12.35 -0.1,12.35
  pour Route3 (isolate 0.254, rank 3, no thermals): -0.25,12.05 6.12,12.05 8.2,9.8 37.4,9.95 37.55,-0.55 -0.25,-0.55
  pour Bottom (isolate 0.254, rank 2, no thermals): 34.5,0.25 34.5,11 36.25,12.75 48.25,13 48.25,0.5
  pour Route3 (isolate 0.254, rank 2, no thermals): 48.25,12.75 48.25,0 34.5,0 34.5,11 36.25,12.75
  pour Top (isolate 0.254, rank 2, no thermals): 40.75,17.75 45.5,17.75 45.5,9 40.75,9
BOOT
  Top 0.16: C4.2 7.79,26.34 7.79,24.2 8.63,23.36 U$1.44
CAN_RX  (via drill 0.3)
  Top 0.16: U$3.59 28.28,20.6 | 28.28,20.6 27.3,19.62 v26.66,19.62 | U$6.4 24.88,17.24 v24.9,17.06 | U$3.61 29.28,20.48 29.22,20.42 28.46,20.42 28.28,20.6
  Bottom 0.16: v24.9,17.06 24.9,18.5 26.02,19.62 v26.66,19.62
CAN_TX
  Top 0.16: U$3.62 29.78,22.58 29.22,23.14 28.42,23.14 27.78,22.5 U$3.58 27.78,20.58 27.46,20.26 26.28,20.26 U$6.1
CANH
  Top 0.16: U$6.7 30.21,18.36 30.6,18.75 34,18.75 40.25,25 CAN.P$2
CANL
  Top 0.16: U$6.6 30.31,17.86 30.7,18.25 34,18.25 38.25,22.5 CAN.P$1
CPH
  Top 0.16: C5.1 5.64,16.37 5.86,16.58 5.86,18.82 6.02,18.98 7.46,18.98 U$1.4
CPL
  Top 0.16: U$1.3 7.96,20.12 7.14,19.3 5.86,19.3 5.22,18.66 5.22,18.3 C5.2
CS  (via drill 0.3)
  Top 0.16: v17.15,20.6 17.6,20.15 20.54,20.15 20.81,20.42 23.46,20.42 23.78,20.74 U$3.50
  Bottom 0.16: v17.15,20.6 17.15,20.57 U$11.5
DEVICE3.3
  Top 0.16: U$1.36 12.11,26.83 C7.1
ENABLE  (via drill 0.3)
  Top 0.16: U$3.44 21.32,25.25 21.37,25.3 v22.83,25.3 | U$1.42 8.43,24.95 v8.54,24.8 | U$1.38 10.74,25.45 10.34,25.85 v10.34,26.6 | U$1.40 8.99,25.79 v8.99,26.15 | U$1.33 | U$1.33 13.86,25.38 13.86,25.59 v14.12,25.85
  Bottom 0.16: v10.34,26.6 10.19,26.75 9.74,26.75 9.14,26.15 v8.99,26.15 8.96,26.18 8.1,26.18 7.79,25.87 7.79,24.95 7.94,24.8 v8.54,24.8 8.8,25.06 12.42,25.06 13.21,25.85 v14.12,25.85 14.45,26.18 21.54,26.18 22.42,25.3 v22.83,25.3
FAULT
  Top 0.16: U$1.28 15.46,23.46 16.42,23.46 17.86,24.9 18.5,24.9 19.38,25.78 R4.1
FB
  Top 0.16: U$1.1 7.26,20.86 6.34,19.94 6.02,19.94 5.06,18.98 3.62,18.98 R1.1 3.37,18.21 R2.2
GHA
  Top 0.16: U$1.8 9.22,17.9 9.22,17.22 7.94,15.94 7.94,11.8 6.22,10.08 6.22,5.55 6.12,5.15 Q1.4
GHB
  Top 0.16: Q3.4 22.18,4.26 23.1,5.22 23.1,14.66 22.26,15.46 16.9,15.46 15.3,17.06 14.9,17.06 U$1.17
GHC
  Top 0.16: U$1.18 15.3,17.38 15.46,17.38 17.06,15.78 22.5,15.78 22.82,15.46 28.42,15.46 28.74,15.14 28.74,5.03 Q5.4
GLA
  Top 0.16: Q2.4 7.25,9.3 7.25,10.1 8.58,11.43 8.58,15.62 9.86,16.9 9.86,17.06 10.44,17.64 U$1.10
GLB
  Top 0.16: U$1.15 12.88,17.72 13.54,17.06 13.54,16.42 12.74,15.62 12.74,9.4 Q4.4
GLC
  Top 0.16: Q6.4 29.38,11.18 29.38,15.46 28.74,16.1 23.14,16.1 22.82,16.42 17.7,16.42 U$1.20
GND  (via drill 0.3)  (5 unrouted)
  Top 0.16: 10.7,13.1 10.7,14.1 R7.1 10.8,12.88 10.66,12.74 9.38,12.74 9.22,12.9 9.22,15.3 10.5,16.58 10.7,16.58 U$1.12 | U$1.43 11.25,21.41 U$1.49 | U$1.2 8.41,21.41 U$1.49 | U$1.27 14.39,21.71 14.39,21.5 | U$1.49 11.61,24.61 U$1.35 13.38,26.38 C7.2 | v22.82,23.15 22.18,23.79 U$3.47 20.57,23.79 19.94,24.42 19.56,24.42 C32.2 | U$3.12 31.6,28.79 v31.36,28.55 | v31.07,31.25 30.28,32.04 U$3.18 30.28,34.42 C27.2 30.81,34.95 LED2.C | U$3.31 23.78,31.94 v24.02,31.7 | U$6.9 26.61,18.36 U$6.2 24.39,18.36 C34.2 | U$6.9 26.86,17.94 v26.26,18.06 | U$3.60 28.78,22.29 v28.67,22.4 | 14.98,19.78 14.98,19.94 15.24,20.2 U$1.22 U$1.21 18.06,16.74 22.98,16.74 23.3,16.42 28.9,16.42 29.7,15.62 29.7,12.42 30.02,12.1 30.75,12.1 v30.9,11.95 | 15.77,13.45 15.46,13.46 15.46,12.9 15.3,12.74 13.7,12.74 13.7,15.14 14.02,15.46 15.46,15.46 v15.77,15.77 v15.77,15.78 | C18.2 18.8,18.2 U$11.TH | v30.34,23.36 30.28,23.3 U$3.63 30.28,19.94 C33.2 | v32.82,22.38 34.29,22.38 C31.2 35.54,22.4 C10.2 | XT1.2 34.65,26.85 v34.62,26.88 | C41.2 34.45,31.93 v34.36,32.02 | U$6.8 27.61,18.86 U$6.9 | 17.72,30.02 LED1.C | U$1.13 12.14,16.77 v11.15,15.78 | R27.1 17.45,29.75 LED1.C | v1.05,17.09 1.52,17.09 R2.1 | v18.76,22.19 18.71,22.24 VREFCAP.2 | YCAP1.1 v3.46,31.94 | v33.3,10.75 34.18,9.87 34.18,6.94 YCAP2.1 | 12.12,30.91 C19.2 9.95,30.91 v9.91,30.87 | v17.7,33.22 17.7,32.01 PROG.3 17.61,32.01 LED1.C
  Top 0.26: D1.A 2.2,24.05 | 1.32,30.71 C3.2
  Top 0.3: 2.2,24.05 C2.2
  Top 0.305: D1.A 1.44,24.1 0.9,24.1 0.42,24.58 0.42,30.02 1,30.6 v1.25,30.6 | C17.2 1.66,21.41 C2.2 | v8.2,29.41 7.94,28.71
  Top 0.406: 30.95,12.8 v30.9,12.55 | MC1.2 5.48,29.7 LDFM33PUR.4 8.1,29.7 LDFM33PUR.EXP
  Top 1.016: C16.2 30.95,12.8
  Route3 0.16: v22.82,23.15 22.67,23.15 22.82,23 | v32.82,22.38 33.13,22.15 | v31.07,31.25 31.37,31.1 | v24.02,31.7 24.17,31.7 | v26.26,18.06 26.26,17.91 | v28.67,22.4 28.52,22.55 | v30.34,23.36 30.19,23.51 | CAN.P$3 42,27.5 37,22.5
  Route3 0.813: 6.72,16.74 6.72,14.5
  Bottom 0.16: 8.15,14.9 7.85,14.45 | 18.2,18.95 18.35,19.1 U$11.TH 19.25,19.25 U$11.8 | v11.15,15.78 11.46,15.78 11.78,15.46 15.45,15.46 v15.77,15.78
  other vias: 33.3,11.95 9.91,13.45 8.69,21.35 32.7,11.95 32.1,11.95 31.5,11.95 31.5,12.55 32.1,12.55 32.7,12.55 33.3,12.55 18.17,14.8 16.53,13.45 14.73,13.45 16.53,14.05 15.93,14.05 15.33,14.05 14.73,14.05 14.73,14.65 15.33,14.65 15.93,14.65 16.53,14.65 11.71,13.45 11.71,14.05 11.11,14.05 10.51,14.05 9.91,14.05 9.91,14.65 10.51,14.65 11.11,14.65 11.71,14.65 0.6,14.8 11.69,18.35 14.69,21.35 11.54,24.35 10.19,22.85 13.19,19.85 11.69,21.35 13.04,22.85 10.19,19.85 30.9,11.35 31.5,11.35 32.1,11.35 32.7,11.35 33.3,11.35 32.7,10.75 32.1,10.75 31.5,10.75 30.9,10.75 1.5,14.8 2.4,14.8 3.3,14.8 4.2,14.8 5.1,14.8 6,14.8 0.6,13.3 1.5,13.3 2.4,13.3 3.3,13.3 4.2,13.3 5.1,13.3 6,13.3 18.17,13.3 19.07,14.8 19.97,14.8 20.87,14.8 21.77,14.8 19.07,13.3 19.97,13.3 20.87,13.3 21.77,13.3 24.17,14.8 25.07,14.8 25.97,14.8 26.87,14.8 27.77,14.8 24.17,13.3 25.07,13.3 25.97,13.3 26.87,13.3 27.77,13.3 18.5,18.5 46.25,17.4 46.25,16.2 46.25,15 46.25,13.8
  pour Route3 (isolate 0.254, no thermals): -0.5,15.9 10.4,15.9 10.4,17 16.51,17 16.51,15.95 30,16 32,18.15 37.25,18.15 37.5,37.5 -0.5,37.5
  pour Top (isolate 0.254, rank 2, no thermals): 14.32,13.21 16.87,13.21 16.87,15.05 14.32,15.05
  pour Top (no thermals): 17.77,15.05 22.27,15.05 22.27,12.65 17.77,12.65
  pour Top (no thermals): 23.45,12.65 28.56,12.65 28.56,15.05 23.45,15.05
  pour Top (isolate 0.254, no thermals): -0.25,15.18 6.35,15.18 6.35,12.95 -0.25,12.95
  pour Top (isolate 0.254, rank 2, no thermals): 30.55,12.8 33.81,12.8 33.81,9.65 30.5,9.65
  pour Route3 (rank 3, no thermals): -0.25,15.05 37.25,15.05 37.1,10.25 8.44,10.1 6.2,12.65 -0.25,12.65
  pour Top (isolate 0.254, rank 2, no thermals): 12.37,13.1 12.37,15.05 9.66,15.05 9.66,13.1
  pour Route2 (isolate 0.254, rank 4, no thermals): 0.2,15.05 36.8,15.05 36.8,10.1 0.2,10.1
  pour Bottom (isolate 0.305, rank 2, no thermals): 7.34,24.8 13.79,24.8 15.44,23.15 15.44,17.9 14.84,17.3 7.49,17.3 6.59,18.2 6.59,24.05
  pour Bottom (isolate 0.254, rank 2, no thermals): 0.25,15 30.25,15 32.5,17.5 48.25,17.75 48.25,13.5 36,13.25 34,11.25 34,10.25 19.5,10.25 17.25,12.5 0.25,12.5
  pour Route3 (isolate 0.254, rank 2, no thermals): 48.25,17.5 48.25,13.25 34.75,13.25 30.25,13.75 30.5,15.25 32.5,17.5
  pour Route2 (isolate 0.254, rank 2, no thermals): 48.25,17.5 48.25,13.25 34.75,13.25 30.25,13.5 30.5,15.25 32.5,17.5
  pour Top (isolate 0.254, rank 2, no thermals): 46,17.75 48.25,17.75 48.25,9 46,9
  pour Top (isolate 0.254, rank 2, no thermals): 40.25,17.75 40.25,9 38,9 38,13.25 35,13.25 35,17.75
I_A  (via drill 0.3)
  Top 0.16: v29.62,26.7 30.62,26.7 30.71,26.79 U$3.8 | U$1.25 16.38,21.9 v16.46,21.82
  Bottom 0.16: v29.62,26.7 28.82,26.7 24.62,22.5 23.62,22.5 22.66,21.54 16.74,21.54 v16.46,21.82
I_B  (via drill 0.3)
  Top 0.16: U$3.9 30.38,27.29 v30.32,27.35 | v20.21,22.13 19.3,21.22 16.34,21.22 U$1.24
  Bottom 0.16: v30.32,27.35 28.97,27.35 28.67,27.05 27.97,26.3 24.47,22.85 23.38,22.85 22.82,22.25 20.33,22.25 v20.21,22.13
INDICATOR
  Top 0.16: U$3.25 26.78,35.43 R22.2
MCO
  Top 0.16: U$3.5 34.82,25.29 XT1.1
MISO  (via drill 0.3)
  Top 0.16: U$3.52 24.78,20.62 23.78,19.62 22.31,19.62 v21.77,19.08
  Bottom 0.16: U$11.7 18.8,20.02 18.8,20.6 18.95,20.75 21.47,20.75 21.77,20.45 v21.77,19.08
MOSI  (via drill 0.3)
  Top 0.16: U$3.53 25.28,20.64 23.94,19.3 22.66,19.3 22.34,18.98 22.34,17.43 v22.21,17.3
  Bottom 0.16: v22.21,17.3 22.21,16.4 21.91,16.1 16.7,16.1 16.25,16.55 16.25,19.1 16.4,19.25 U$11.4
N$1
  Top 0.16: LED1.A 19.37,28.77 R5.1
N$2
  Top 0.16: CHOKE.2 35.57,29.51 C41.1 34.23,29.29 U$3.13
N$3
  Top 0.16: U$3.30 24.28,33.88 C9.2
N$4  (via drill 2.1 pad 3.8)
  Top 0.16: YCAP1.2 1.26,34.26 v2,35
N$5  (via drill 2.1 pad 3.8)
  other vias: 35,35
N$6  (via drill 2.1 pad 3.8)
  Top 0.16: YCAP2.2 34.98,2.02 v35,2 36.1,3.1 YCAP3.2
N$7  (via drill 2.1 pad 3.8)
  other vias: 2,2
N$24  (via drill 0.3)
  Top 0.16: U$3.14 28.26,29.79 27.33,28.86 26.28,28.86 v25.81,28.87 | R26.1 16.55,28.07 R27.2 v15.16,28.45
  Bottom 0.16: v25.81,28.87 25.81,28.69 24.9,27.78 22.34,27.78 22.02,27.46 16.15,27.46 v15.16,28.45
N$28
  Top 0.16: LED2.A 27.69,35.88 R22.1
N$30
  Top 0.16: XT1.3 34.29,28.05 33.86,27.62 33.86,26.02 33.63,25.79 U$3.6
NRST  (via drill 0.3)
  Top 0.16: U$3.7 31.73,26.29 v31.46,26.02 | v15.78,33.7 15.78,32.05 PROG.5
  Bottom 0.16: v31.46,26.02 31.46,26.34 32.42,27.3 32.42,30.98 28.26,35.14 17.22,35.14 v15.78,33.7
PHASA  (via drill 0.3)
  Top 0.16: U$1.9 9.54,17.54 9.54,17.06 8.26,15.78 8.26,11.64 6.54,9.92 6.54,7.49 7.08,7.4 7.11,7.4
  other vias: 10.86,5.3 10.86,5.9 10.86,6.5 10.86,7.1 10.86,7.7 7.26,5.3 7.26,5.9 7.26,6.5 7.26,7.1 7.26,7.7 7.86,5.3 7.86,5.9 7.86,6.5 7.86,7.1 7.86,7.7 8.46,5.3 8.46,5.9 8.46,6.5 8.46,7.1 8.46,7.7 9.06,5.3 9.06,5.9 9.06,6.5 9.06,7.1 9.06,7.7 9.66,5.3 9.66,5.9 9.66,6.5 9.66,7.1 9.66,7.7 10.26,5.3 10.26,5.9 10.26,6.5 10.26,7.1 10.26,7.7 7.26,4.7 7.86,4.7 8.46,4.7 9.06,4.7 9.66,4.7 10.26,4.7 10.86,4.7 2,5.31 2.6,5.31 3.2,5.31 3.8,5.31 4.4,5.31 4.4,4.71 3.8,4.71 3.2,4.71
  pour Top (isolate 0.254, no thermals): 1.75,5.72 5.15,5.72 5.15,4.25 6.62,4.25 6.62,7.95 11.71,7.95 11.75,5.85 12.2,5.45 12.2,0.45 1.75,0.3
  pour Route2 (isolate 0.254, no thermals): 1.75,5.88 6.79,5.88 6.79,8.12 11.85,8.12 11.8,0.45 1.75,0.3
PHASB  (via drill 0.3)
  Top 0.16: Q4.5 14.85,6.4 13.56,8 13.56,10.17 13.06,10.67 13.06,15.46 13.86,16.26 13.86,17.38 13.2,18.04 U$1.16
  other vias: 12.95,5.15 12.95,5.75 12.95,6.35 12.95,6.95 12.95,7.55 13.55,5.15 13.55,5.75 13.55,6.35 13.55,6.95 13.55,7.55 14.15,5.15 14.15,5.75 14.15,6.35 14.15,6.95 14.15,7.55 14.75,5.15 14.75,5.75 14.75,6.35 14.75,6.95 14.75,7.55 15.35,5.15 15.35,5.75 15.35,6.35 15.35,6.95 15.35,7.55 15.95,5.15 15.95,5.75 15.95,6.35 15.95,6.95 15.95,7.55 16.55,5.15 16.55,5.75 16.55,6.35 16.55,6.95 16.55,7.55 12.95,4.55 13.55,4.55 14.15,4.55 14.75,4.55 15.35,4.55 15.95,4.55 16.55,4.55 18.35,4.85 18.95,4.85 19.55,4.85 20.15,4.85 20.75,4.85 18.35,4.25 18.95,4.25 19.55,4.25 20.15,4.25 20.75,4.25
  pour Top (isolate 0.254, rank 2, no thermals): 12.65,7.65 12.65,3.95 12.61,3.95 12.61,0.3 21.45,0.3 21.45,5.35 17.05,5.35 17.05,7.65
  pour Route2 (isolate 0.254, rank 2, no thermals): 12.36,8.12 12.36,3.95 12.31,3.95 12.31,0.3 21.45,0.3 21.45,5.37 17.2,5.37 17.2,8.12
PHASC  (via drill 0.3)
  Top 0.16: v29.76,9.05 29.06,9.46 29.06,15.3 28.58,15.78 22.98,15.78 22.66,16.1 17.3,16.1 U$1.19
  other vias: 33.36,9.05 33.36,8.45 33.36,7.85 33.36,7.25 33.36,6.65 32.76,9.05 32.76,8.45 32.76,7.85 32.76,7.25 32.76,6.65 29.76,8.45 29.76,7.85 29.76,7.25 29.76,6.65 30.36,9.05 30.36,8.45 30.36,7.85 30.36,7.25 30.36,6.65 30.96,9.05 30.96,8.45 30.96,7.85 30.96,7.25 30.96,6.65 31.56,9.05 31.56,8.45 31.56,7.85 31.56,7.25 31.56,6.65 32.16,9.05 32.16,8.45 32.16,7.85 32.16,7.25 32.16,6.65 26.61,4.4 26.01,4.4 25.41,4.4 24.81,4.4 24.21,4.4 24.21,3.8 24.81,3.8 25.41,3.8 26.01,3.8 26.61,3.8
  pour Top (isolate 0.254, no thermals): 23.57,5.05 23.57,0.35 33.97,0.35 33.97,9.85 28.3,9.85 28.3,3.15 27.22,3.15 27.22,5.05
  pour Route2 (isolate 0.254, no thermals): 23.57,5.22 23.57,0.35 33.97,0.35 33.97,9.56 29.1,9.56 29.1,5.22
PWMA  (via drill 0.3)
  Top 0.16: U$1.41 8.55,25.55 v8.39,25.55 | 23.99,26.15 v24.02,26.15 23.81,25.94 22.26,25.94 22.11,25.79 U$3.43
  Bottom 0.16: v8.39,25.55 8.56,25.38 10.82,25.38 11.94,26.5 21.7,26.5 22.34,25.86 23.62,25.86 23.91,26.15 v24.02,26.15
PWMB  (via drill 0.3)
  Top 0.16: U$3.42 22.98,26.29 v23.27,26.6 | U$1.39 9.65,25.85 v9.79,26
  Bottom 0.16: v9.79,26 9.88,25.86 10.82,25.86 11.78,26.82 21.86,26.82 22.34,26.34 22.82,26.34 23.08,26.6 v23.27,26.6
PWMC  (via drill 0.3)
  Top 0.16: U$3.41 22.26,26.79 v22.52,27.05 | U$1.37 11.09,25.93 v11.09,26.9
  Bottom 0.16: v11.09,26.9 11.33,27.14 22.02,27.14 22.11,27.05 v22.52,27.05
SCK  (via drill 0.3)
  Top 0.16: v21.18,18.19 21.17,18.34 21.17,19.57 21.54,19.94 23.62,19.94 24.26,20.58 24.26,21.27 U$3.51
  Bottom 0.16: v21.18,18.19 20.74,17.75 U$11.12
SPA  (via drill 0.3)
  Top 0.16: 10.33,11.28 R7.2 10.7,11.15 10.7,12.3 10.58,12.42 9.22,12.42 8.9,12.74 8.9,15.46 U$1.11 | 10.33,11.28 10.1,11.4 | 10.33,11.29 10.33,11.28
  other vias: 9.35,10.4 9.95,10.4 10.55,10.4 11.15,10.4 11.75,10.4 11.75,11 11.15,11 10.55,11 9.95,11 9.35,11
  pour Top (isolate 0.254, rank 2, no thermals): 7.86,8.6 12.21,8.6 12.21,12.05 7.86,12.05
  pour Bottom (isolate 0.254): 6.82,12.1 12.74,12.1 12.74,10.18 8.74,10.18
SPB  (via drill 0.3)
  Top 0.16: R6.2 15.4,11.36 15.46,12.26 15.3,12.42 13.38,12.42 13.38,15.3 13.86,15.78 14.98,15.78 15.14,15.94 15.14,16.3 v15.16,16.32 | U$1.14 12.6,17.36 13.06,16.9 13.06,16.86 v12.28,16.08
  Bottom 0.16: v15.16,16.32 15.06,16.42 12.62,16.42 v12.28,16.08
  other vias: 14.45,10.4 15.05,10.4 15.65,10.4 16.25,10.4 16.85,10.4 16.85,11 16.25,11 15.65,11 15.05,11 14.45,11
  pour Top (isolate 0.254, rank 2, no thermals): 17.3,12.06 14,12.06 14,8.75 17.3,8.75
  pour Bottom (isolate 0.254): 13.38,12.1 16.74,12.1 18.66,10.18 13.38,10.18
SPI-MISO  (via drill 0.3)
  Top 0.16: U$3.22 28.28,31.62 v28.22,31.56 | R3.1 18.07,25.59 17.73,25.59 v16.81,24.67 16.81,24.33 16.26,23.78 15.1,23.78 U$1.29
  Bottom 0.16: v28.22,31.56 28.22,29.45 27.94,29.02 27.94,26.77 24.95,23.78 22.02,23.78 20.9,24.9 17.04,24.9 v16.81,24.67
SPI-MOSI  (via drill 0.3)
  Top 0.16: U$3.23 27.78,32.02 27.62,31.86 v27.62,30.96 | v15.77,24.34 15.93,24.41 15.62,24.1 14.7,24.1 U$1.30
  Bottom 0.16: v27.62,30.96 27.62,26.98 24.74,24.1 22.18,24.1 21.06,25.22 16.49,25.22 v15.77,24.34
SPI-NSS-DRV  (via drill 0.3)
  Top 0.16: U$3.20 29.28,31.26 27.62,29.6 v26.42,29.6 | v14.88,25.57 14.73,25.57 U$1.32
  Bottom 0.16: v14.88,25.57 15.17,25.86 21.38,25.86 22.5,24.74 24.42,24.74 26.82,27.14 26.82,29.22 26.44,29.6 v26.42,29.6
SPI-SCK  (via drill 0.3)
  Top 0.16: U$3.21 28.78,31.21 27.77,30.2 v27.02,30.2 | v15.62,25.25 15.62,25.06 14.98,24.42 14.3,24.42 U$1.31
  Bottom 0.16: v15.62,25.25 15.91,25.54 21.22,25.54 22.34,24.42 24.58,24.42 27.3,27.14 27.3,29.7 27.02,29.98 v27.02,30.2
SW
  Top 0.26: 6.63,24.63 D1.C 6.39,24.62 | C4.1 6.06,26.98
  Top 0.3: U$1.45 6.63,24.63
  pour Top (no thermals): 1.54,26.98 6.18,26.98 6.18,23.46 4.74,23.46 4.74,25.54 1.54,25.54
TCK  (via drill 0.3)
  Top 0.16: U$3.49 23.28,22.71 25.07,24.5 25.07,27.65 v23.42,29.3 | v18.83,31.1 18.74,31.1 PROG.2
  Bottom 0.16: v23.42,29.3 20.63,29.3 v18.83,31.1
TMS  (via drill 0.3)
  Top 0.16: U$3.46 23.96,24.29 24.62,24.95 24.62,27.35 23.27,28.7 v22.65,28.7 | v16.83,31.1 16.74,31.1 PROG.4
  Bottom 0.16: v22.65,28.7 19.23,28.7 v16.83,31.1
USART_RX  (via drill 0.3)
  Top 0.16: v31.62,33.86 31.62,33.63 U$3.17 | PROG.7 v13.73,33.81
  Bottom 0.16: v13.73,33.81 15.97,36.05 29.43,36.05 v31.62,33.86
USART_TX  (via drill 0.3)
  Top 0.16: v32.87,31.55 32.87,30.88 U$3.16 | PROG.6 14.67,32.01 v14.67,33.77
  Bottom 0.16: v32.87,31.55 32.72,31.7 32.31,31.7 28.39,35.62 16.52,35.62 v14.67,33.77
VCP
  Top 0.16: C6.2 7.34,18.18 U$1.5

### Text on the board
tNames: HKC Integrated / V2.2 / Ben Katz / 10/18 | :P | - | + | U | V | W

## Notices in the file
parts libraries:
SparkFun-Aesthetics: Licensing: Creative Commons ShareAlike 4.0 International - https://creativecommons.org/licenses/by-sa/4.0
inductor-bourns: Copyright (C) 2008, Bob Starr
